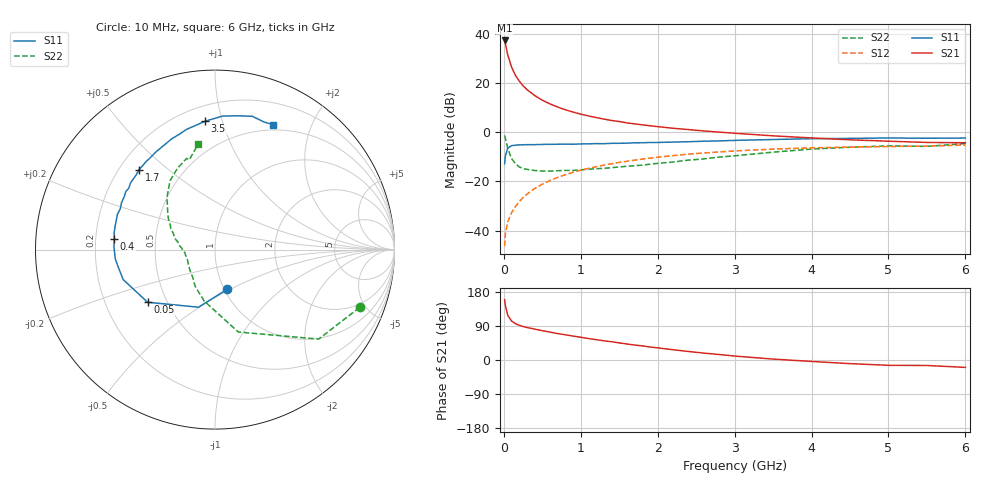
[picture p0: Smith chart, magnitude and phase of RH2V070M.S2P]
! SIEMENS Small Signal Semiconductors
! BFR106
! Si NPN RF Bipolar Junction Transistor in SOT23
! VCE = 2 V  IC = 70 mA
! Common Emitter S-Parameters:  August  1996
# GHz  S  MA  R  50
!  f  S11  S21  S12  S22
! GHz  MAG  ANG  MAG  ANG  MAG  ANG  MAG  ANG
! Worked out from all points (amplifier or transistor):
!   36 points, 10 MHz to 6 GHz, reference 50 ohm
!   highest |S21| = 37.5 dB at 10 MHz (marker M1)
!   |S21| within 3 dB of that: start of sweep to 31.39 MHz
!   unconditionally stable (mu >= 1): 189.5 MHz to 2.865 GHz; 5.053 GHz to end of sweep
!   at 250 MHz: K = 1.05, MAG = 21.5 dB, |S12| = -26.6 dB
!   at 1.4 GHz: K = 1.07, MAG = 7.3 dB, |S12| = -12.8 dB
!   at 6 GHz: K = 1.01, MAG = -0.1 dB, |S12| = -5.1 dB
!   S11 on the Smith chart (normalised r, x): 10 MHz: 1.03, -0.48; 50 MHz: 0.39, -0.30; 400 MHz: 0.28, +0.05; 1.7 GHz: 0.28, +0.40; 3.5 GHz: 0.30, +0.88; 6 GHz: 0.44, +1.48
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0.01  0.2314 -72.9  75.04 159.5  0.0048 78.4  0.8676 -21.8
0.02  0.3338 -106.0  64.54 143.8  0.0086 66.8  0.7631 -40.8
0.05  0.4765 -142.0  38.66 118.3  0.0149 58.2  0.4772 -74.2
0.1  0.5381 -161.9  21.57 103.0  0.023 63.5  0.2927 -101.9
0.15  0.5493 -170.6  14.69 95.9  0.0306 66.8  0.2325 -118.5
0.2  0.5582 -174.8  11.18 91.6  0.0387 69.5  0.1983 -128.7
0.25  0.5601 -178.7  8.934 88.3  0.047 71.0  0.1834 -138.4
0.3  0.5631 178.7  7.487 85.8  0.0552 72.4  0.1766 -143.8
0.4  0.5644 173.9  5.668 81.5  0.0717 72.6  0.1676 -153.4
0.5  0.57 170.2  4.549 77.4  0.0881 72.0  0.1633 -159.7
0.6  0.5719 166.3  3.816 73.6  0.1046 71.2  0.1628 -163.6
0.7  0.5744 162.7  3.298 69.7  0.1211 69.9  0.1659 -167.2
0.9  0.5745 156.7  2.603 63.2  0.154 67.0  0.1681 -174.1
1.1  0.5849 149.9  2.167 56.7  0.185 64.0  0.1783 -177.9
1.3  0.5897 144.5  1.871 50.7  0.2156 60.6  0.1856 177.4
1.7  0.6148 133.5  1.493 39.5  0.2724 53.8  0.2099 169.0
2.2  0.6358 121.2  1.217 27.1  0.3372 45.1  0.2493 158.9
3  0.6883 103.3  0.962 10.4  0.4194 31.7  0.3339 142.0
3.5  0.7174 94.4  0.853 2.4  0.458 24.0  0.396 132.5
4.5  0.7562 80.3  0.708 -9.6  0.5015 9.8  0.499 114.8
5.5  0.7616 68.9  0.625 -14.5  0.5267 1.2  0.5199 106.0
6  0.768 65.0  0.616 -19.5  0.5539 -5.5  0.5938 99.2
